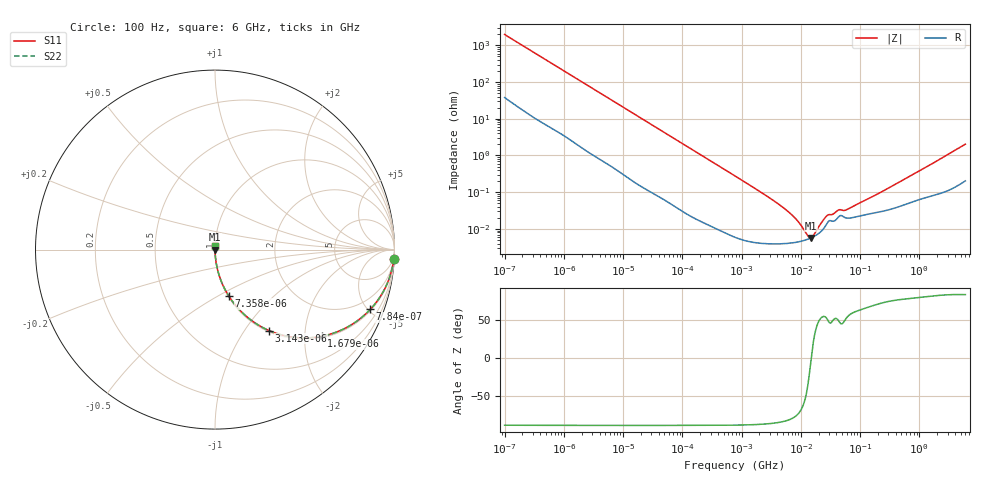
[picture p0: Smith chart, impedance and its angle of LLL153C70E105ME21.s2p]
!Murata Part Number: LLL153C70E105ME21
!These Parameters are Measured in Series Mode Connection
!Data Generated on Mar 13, 2026
!  o--ll--o
!Port1  Port2
!  o------o
!Operation Temp=25[degC], DC Bias Voltage=0[V]
!Freq. Start=100[Hz] Stop=6[GHz] 401[Steps]
# Hz S RI R 50
!Freq.(Hz) S11(Real) S11(Imag) S21(Real) S21(Imag) S12(Real) S12(Imag) S22(Real) S22(Imag)
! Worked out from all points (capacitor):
!   401 points, 100 Hz to 6 GHz, reference 50 ohm
!   read as one part in series: C = 801 nF near 109 Hz
!   lowest |Z| = 5.69 mohm at 14.88 MHz (marker M1)
!   series resonance near 14.98 MHz, so ESL is about 140 pH
!   S11 on the Smith chart (normalised r, x): 100 Hz: 2, -40; 784 Hz: 1.09, -5.16; 1.679 kHz: 1.04, -2.43; 3.143 kHz: 1.02, -1.31; 7.358 kHz: 1.01, -0.56; 6 GHz: 1.00, +0.04
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100  0.9965 -0.0503  0.0035 0.0503  0.0035 0.0503  0.9965 -0.0503
293  0.9768 -0.1425  0.0232 0.1425  0.0232 0.1425  0.9768 -0.1425
784  0.8651 -0.3331  0.1349 0.3331  0.1349 0.3331  0.8651 -0.3331
1679  0.5949 -0.4829  0.4051 0.4829  0.4051 0.4829  0.5949 -0.4829
2008  0.5088 -0.4921  0.4912 0.4921  0.4912 0.4921  0.5088 -0.4921
3143  0.3019 -0.4514  0.6981 0.4514  0.6981 0.4514  0.3019 -0.4514
4702  0.165 -0.3635  0.835 0.3635  0.835 0.3635  0.165 -0.3635
7358  0.0767 -0.2587  0.9233 0.2587  0.9233 0.2587  0.0767 -0.2587
15752  0.0189 -0.1296  0.9811 0.1296  0.9811 0.1296  0.0189 -0.1296
40335  0.00345 -0.0519  0.9965 0.0519  0.9965 0.0519  0.00345 -0.0519
774597  6.67e-05 -0.00277  0.9999 0.00277  0.9999 0.00277  6.67e-05 -0.00277
4856642  3.96e-05 -0.000398  1 0.000398  1 0.000398  3.96e-05 -0.000398
7266822  4.17e-05 -0.000227  1 0.000227  1 0.000227  4.17e-05 -0.000227
1.137099e7  4.85e-05 -8.03e-05  1 8.03e-05  1 8.03e-05  4.85e-05 -8.03e-05
1.487547e7  5.69e-05 -2e-06  0.9999 2e-06  0.9999 2e-06  5.69e-05 -2e-06
1.555665e7  5.89e-05 1.09e-05  0.9999 -1.09e-05  0.9999 -1.09e-05  5.89e-05 1.09e-05
1.946e7  7.27e-05 7.68e-05  0.9999 -7.68e-05  0.9999 -7.68e-05  7.27e-05 7.68e-05
2.911731e7  0.000159 0.000184  0.9998 -0.000184  0.9998 -0.000184  0.000159 0.000184
4.35672e7  0.000214 0.00025  0.9998 -0.00025  0.9998 -0.00025  0.000214 0.00025
6.233367e7  0.000196 0.000286  0.9998 -0.000286  0.9998 -0.000286  0.000196 0.000286
3.124326e8  0.000336 0.00129  0.9997 -0.00129  0.9997 -0.00129  0.000336 0.00129
6e9  0.00244 0.0202  0.9976 -0.0202  0.9976 -0.0202  0.00244 0.0202
